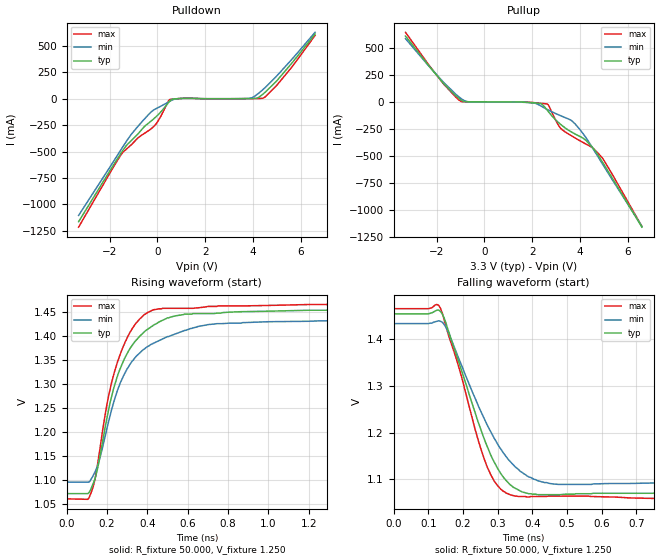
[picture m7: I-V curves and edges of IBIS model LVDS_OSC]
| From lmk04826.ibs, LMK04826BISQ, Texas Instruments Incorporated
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|   Model LVDS
[Model]   LVDS_OSC
Model_type   Output
Polarity   Non-Inverting
Vmeas = 1.25
Vref = 1.25
Cref = 0pF
Rref = 50
|   typ   min   max
|   (nom PVT)   (slow PVT)   (fast PVT)
C_comp   1.2694p   1.2464p   1.3920p
|C_comp (High state)   1.2694p   1.2464p   1.3920p
|C_comp (Low state)   1.7368p   1.7367p   1.7369p
[Voltage Range]   3.3   3.15   3.45
[Temperature Range]   27   125   -40
[Pullup Reference]   3.3   3.15   3.45
[Pulldown Reference]   0   0   -0
[Power Clamp Reference]   3.3   3.15   3.45
[GND Clamp Reference]   0   0   0
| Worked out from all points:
|   slope of the pulldown table from 0 to 0.495 V, typ, clamps not added: 3.84 ohm
|   slope of the pullup table from 0 to 0.495 V, typ, clamps not added: 3.12 kohm
|   falling waveform, R_fixture 50.000, V_fixture 1.250: 20-80 % time 107ps typ, 127ps min, 93.2ps max; typ from 1.46 V to 1.07 V
|   rising waveform, R_fixture 50.000, V_fixture 1.250: 20-80 % time 156ps typ, 191ps min, 131ps max; typ from 1.07 V to 1.46 V
[Pulldown]
|   Voltage   I(typ)   I(min)   I(max)
-3.3V     -1.164A    -1.105A    -1.215A
-1.556V   -525.8mA   -492.8mA   -540.2mA
-1.078V   -393.2mA   -332mA     -432.4mA
-395.3mV  -235mA     -155.4mA   -305.6mA
-84.48mV  -175.9mA   -97.08mA   -246.8mA
521.4mV   -21.65mA   -23.87mA   -7.381mA
1.092V    3.707mA    3.082mA    4.094mA
3.814V    1.636mA    2.314mA    1.277mA
4.133V    3.419mA    33.61mA    1.998mA
4.41V     42.13mA    85.11mA    4.134mA
5.01V     173.2mA    219.4mA    130.8mA
6.598V    611.4mA    628.3mA    598.5mA
[Pullup]
|   Voltage   I(typ)   I(min)   I(max)
-3.3V     611.6mA    587.6mA    646.1mA
-1.712V   173.7mA    183.8mA    169mA
-965.6mV  16.51mA    30.77mA    4.506mA
-684.4mV  1.966mA    2.606mA    2.029mA
2.27V     -11.76mA   -24.81mA   -10.16mA
2.628V    -74.37mA   -68.56mA   -18.92mA
3.19V     -207mA     -126.8mA   -242.4mA
3.674V    -281.4mA   -176.2mA   -316.8mA
4.256V    -356.4mA   -330.7mA   -390.2mA
4.541V    -424mA     -429.7mA   -426.3mA
4.955V    -560.3mA   -577.4mA   -522.1mA
6.598V    -1.161A    -1.153A    -1.154A
[Ramp]
R_load = 50
|   typ   min   max
dV/dt_r   0.230311/1.56545e-10   0.20357/1.9031e-10   0.24665/1.30209e-10
dV/dt_f   0.230311/1.07194e-10   0.20357/1.26958e-10   0.24665/9.33894e-11
[Falling Waveform]
R_fixture = 50.000
V_fixture = 1.250
V_fixture_min = 1.250
V_fixture_max = 1.250
C_fixture = 0.000
|  time   V(typ)   V(min)   V(max)
0s        1.455V     1.434V     1.466V
130ps     1.463V     1.44V      1.473V
155ps     1.425V     1.42V      1.417V
245ps     1.22V      1.256V     1.181V
270ps     1.17V      1.216V     1.126V
300ps     1.123V     1.175V     1.086V
335ps     1.089V     1.139V     1.067V
390ps     1.069V     1.105V     1.062V
475ps     1.067V     1.089V     1.064V
1.99ns    1.071V     1.095V     1.06V
[Rising Waveform]
R_fixture = 50.000
V_fixture = 1.250
V_fixture_min = 1.250
V_fixture_max = 1.250
C_fixture = 0.000
|  time   V(typ)   V(min)   V(max)
0s        1.071V     1.095V     1.06V
110ps     1.073V     1.095V     1.062V
150ps     1.118V     1.126V     1.124V
205ps     1.241V     1.217V     1.27V
250ps     1.315V     1.285V     1.344V
315ps     1.375V     1.342V     1.409V
400ps     1.414V     1.378V     1.449V
535ps     1.442V     1.404V     1.458V
745ps     1.448V     1.426V     1.462V
1.99ns    1.455V     1.434V     1.466V
